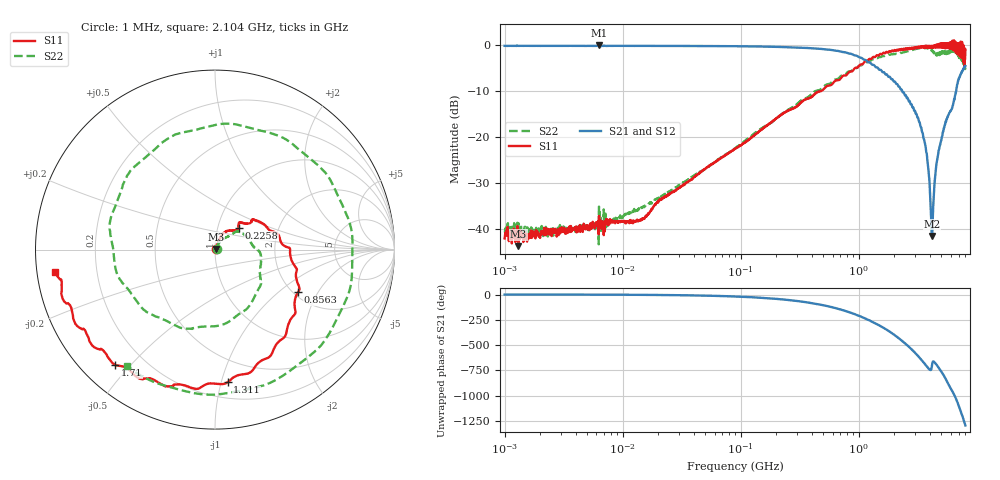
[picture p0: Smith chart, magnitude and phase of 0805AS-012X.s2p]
!s-Parameter Generated by FASTRON Sdn. Bhd.
!FASTRON P/N : 0805AS-012X
!Keysight Technologies: E505271C_MY46733604_B.14.02
!Date: Mon Jun 15 12:48:52 2026
!Version  :Rev01  Mon Jun 15 12:48:52 2026
!Data & Calibration Information:
!Freq  S11:SOLT2(ON)  S21:SOLT2(ON)  S12:SOLT2(ON)  S22:SOLT2(ON)
!PortZ  Port1:50+j0  Port2:50+j0
!When reading reference impedance value at option line is always used.
! Remarks : This data is being provided solely for informational purposes.
# Hz S dB R 50
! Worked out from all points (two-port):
!   1601 points, 1 MHz to 8 GHz, reference 50 ohm
!   highest |S21| = 0.01 dB at 6.301 MHz (marker M1); lowest = -41.5 dB at 4.176 GHz (marker M2)
!   |S21| within 3 dB of the highest: start of sweep to 1.09 GHz
!   lowest |S11| = -43.7 dB at 1.31 MHz (marker M3), VSWR 1.01, Z = 50.5 + j0.378 ohm
!   |S11| at or under -10 dB: start of sweep to 463.6 MHz
!   |S22| runs from -43.3 to -0.3 dB; largest |S21 - S12| = 0.016
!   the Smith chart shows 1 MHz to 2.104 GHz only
!   S11 on the Smith chart (normalised r, x): 1 MHz: 1.02, +0.00; 225.8 MHz: 1.26, +0.32; 856.3 MHz: 2.11, -1.38; 1.311 GHz: 0.32, -1.05; 1.71 GHz: 0.10, -0.45; 2.104 GHz: 0.05, -0.07
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1000000  -42.00 7.5  -0.09 -0.3  -0.08 -0.3  -40.80 6.8
1310238  -43.70 34.9  -0.09 -0.3  -0.08 -0.3  -38.70 -4.9
4479405  -40.20 21.1  -0.10 -1.0  -0.09 -1.1  -39.90 24.2
6301378  -37.10 27.5  0.01 -1.3  0.09 -1.4  -35.10 32.2
2.00676e7  -33.90 54.0  -0.10 -4.5  -0.11 -4.4  -33.30 54.6
8.994653e7  -22.50 65.7  -0.16 -19.7  -0.17 -19.7  -22.40 52.1
2.258311e8  -14.90 42.7  -0.34 -48.5  -0.34 -48.5  -14.80 28.8
4.006501e8  -11.20 36.6  -0.61 -85.3  -0.61 -85.3  -10.50 -31.7
8.562768e8  -5.68 -27.2  -1.81 179.0  -1.81 179.0  -5.61 -151.0
1.310879e9  -2.59 -84.6  -4.22 88.4  -4.22 88.3  -3.01 81.5
1.709681e9  -1.41 -131.0  -6.34 14.2  -6.33 14.1  -2.14 -21.5
1.7949e9  -1.33 -140.0  -6.85 -1.4  -6.84 -1.7  -1.98 -44.2
2.103821e9  -0.92 -172.0  -8.38 -58.2  -8.41 -58.5  -1.81 -127.0
2.63362e9  -0.79 127.0  -11.90 -154.0  -11.90 -154.0  -1.22 99.2
3.029771e9  -0.62 82.7  -14.80 137.0  -14.80 137.0  -0.78 5.0
3.710194e9  -0.45 15.7  -22.90 17.6  -22.80 17.4  -0.49 -170.0
4.176377e9  -0.12 -42.5  -41.50 23.3  -41.50 22.5  -1.03 71.4
4.772513e9  -0.09 -94.7  -22.70 -9.3  -22.70 -9.5  -1.62 -90.2
5.668252e9  -0.42 176.0  -15.50 -155.0  -15.50 -155.0  -1.57 62.9
6.72769e9  0.51 90.5  -9.25 37.2  -9.40 36.7  -0.92 177.0
7.383122e9  -0.09 10.9  -5.92 -91.4  -5.87 -91.6  -2.61 -13.7
8e9  -0.94 -50.4  -4.46 144.0  -4.38 144.0  -4.17 -170.0
